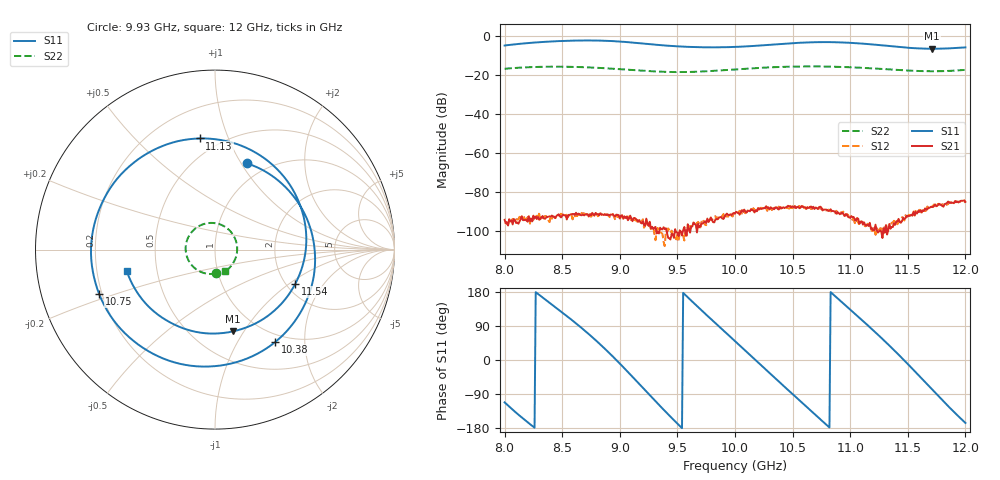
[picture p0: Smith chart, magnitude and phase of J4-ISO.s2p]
!Keysight Technologies,N5234A,MY52241180,A.10.60.03
!Date: Tuesday, May 30, 2023 15:20:48
!Correction: S11(Full 2 Port(1,2))
!S21(Full 2 Port(1,2))
!S12(Full 2 Port(1,2))
!S22(Full 2 Port(1,2))
!S2P File: Measurements: S11, S21, S12, S22:
# Hz S  dB  R 50
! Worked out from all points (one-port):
!   401 points, 8 GHz to 12 GHz, reference 50 ohm
!   lowest |S11| = -6.6 dB at 11.71 GHz (marker M1), VSWR 2.75, Z = 38.4 - j44.7 ohm
!   |S11| at or under -10 dB: nowhere
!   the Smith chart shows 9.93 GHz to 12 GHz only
!   S11 on the Smith chart (normalised r, x): 9.93 GHz: 0.82, +1.06; 10.38 GHz: 0.88, -1.46; 10.75 GHz: 0.19, -0.18; 11.13 GHz: 0.39, +0.79; 11.54 GHz: 2.23, -1.12; 12 GHz: 0.33, -0.11
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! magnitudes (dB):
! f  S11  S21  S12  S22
! 8 GHz  -5.0  -94.4  -96.4  -16.9
! 8.15 GHz  -4.0  -92.6  -92.6  -16.3
! 8.32 GHz  -3.2  -93.3  -92.5  -15.9
! 8.49 GHz  -2.6  -93.2  -91.3  -15.8
! 8.67 GHz  -2.4  -92.1  -91.1  -16.1
! 8.94 GHz  -2.7  -91.5  -91.8  -16.9
! 9.34 GHz  -4.7  -101.4  -100.8  -18.4
! 9.46 GHz  -5.2  -102.0  -102.4  -18.6
! 9.6 GHz  -5.7  -99.3  -98.7  -18.5
! 9.77 GHz  -5.9  -95.4  -95.5  -18.1
! 9.93 GHz  -5.8  -91.3  -91.9  -17.5
! 10 GHz  -5.7  -91.3  -90.9  -17.2
! 10.38 GHz  -4.2  -89.2  -87.7  -16.0
! 10.67 GHz  -3.3  -88.3  -88.8  -15.7
! 10.75 GHz  -3.2  -88.2  -88.6  -15.7
! 10.95 GHz  -3.4  -92.5  -91.9  -16.0
! 11.13 GHz  -4.1  -97.2  -97.6  -16.5
! 11.34 GHz  -5.2  -96.6  -98.6  -17.2
! 11.54 GHz  -6.3  -92.3  -91.7  -17.9
! 11.71 GHz  -6.6  -87.9  -87.7  -18.2
! 11.84 GHz  -6.5  -85.8  -86.7  -18.0
! 12 GHz  -5.9  -85.2  -85.6  -17.5
